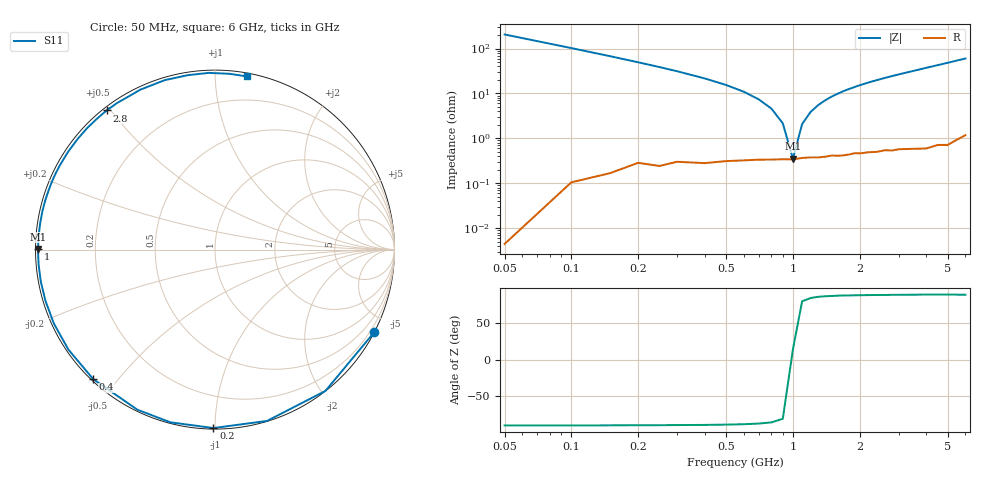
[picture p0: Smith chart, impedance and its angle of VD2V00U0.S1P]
! Infineon Technologies  Discrete & RF Semiconductors
! BBY 55-03
! Si Tuning Diode in SOD323
! VR = 2 V
! S-Parameters:  June  1999
# GHz  S  MA  R  50
!  f  S11
! GHz  MAG  ANG
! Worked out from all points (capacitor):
!   34 points, 50 MHz to 6 GHz, reference 50 ohm
!   read as one part to ground: C = 15.4 pF near 50 MHz
!   lowest |Z| = 354 mohm at 1 GHz (marker M1)
!   series resonance near 996.1 MHz, so ESL is about 1.7 nH
!   S11 on the Smith chart (normalised r, x): 50 MHz: 0.00, -4.12; 200 MHz: 0.01, -0.99; 400 MHz: 0.01, -0.43; 1 GHz: 0.01, +0.00; 2.8 GHz: 0.01, +0.49; 6 GHz: 0.02, +1.20
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0.05  1 -27.3
0.1  0.9992 -52.0
0.15  0.9976 -73.1
0.2  0.9942 -90.5
0.25  0.9939 -104.5
0.3  0.9913 -115.9
0.4  0.9905 -133.2
0.5  0.9886 -145.7
0.6  0.9877 -155.3
0.7  0.9869 -163.1
0.8  0.9867 -169.5
1  0.9864 179.8
1.1  0.9854 175.3
1.3  0.9852 167.4
1.5  0.9839 160.5
1.6  0.9843 157.4
1.8  0.9836 151.5
2  0.9831 146.1
2.2  0.9826 141.1
2.4  0.9828 136.5
2.8  0.9828 127.9
3  0.9822 124.0
3.5  0.9834 115.0
4  0.9848 106.5
4.5  0.9836 98.9
5  0.9852 92.0
5.5  0.9829 85.3
6  0.9809 79.6
